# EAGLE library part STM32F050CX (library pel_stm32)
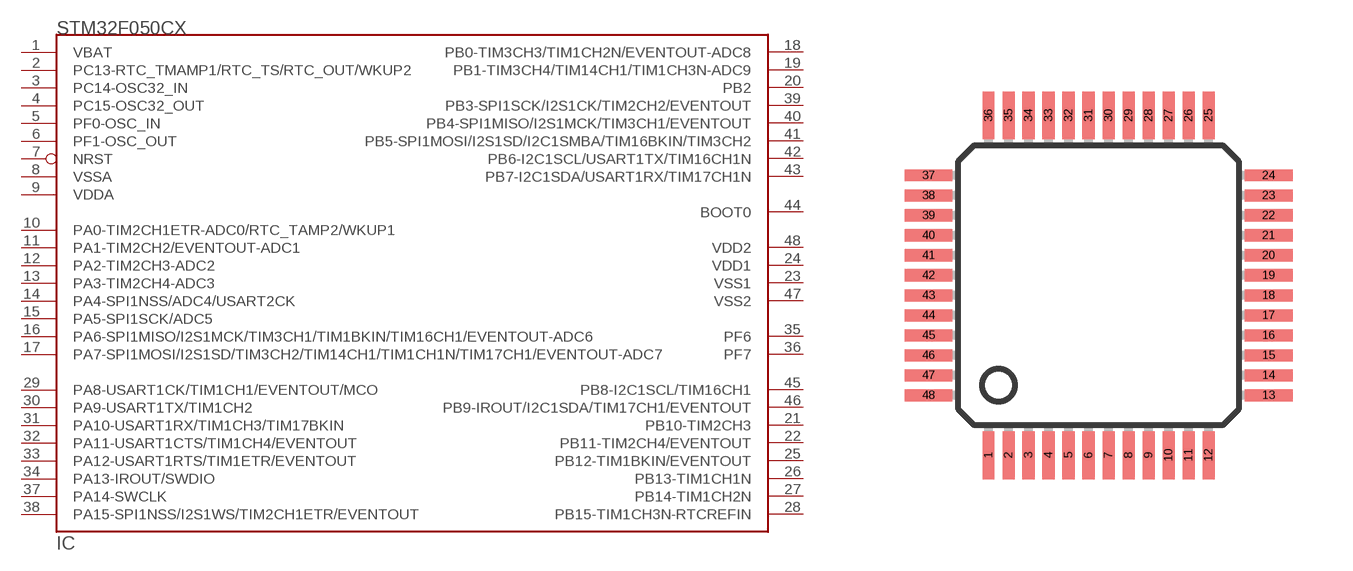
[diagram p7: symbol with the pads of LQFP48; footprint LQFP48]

Designator prefix IC

## STM32F050CX  [LQFP48]
1  VBAT  sup
2  PC13-RTC_TMAMP1/RTC_TS/RTC_OUT/WKUP2
3  PC14-OSC32_IN
4  PC15-OSC32_OUT
5  PF0-OSC_IN  in
6  PF1-OSC_OUT  out
7  NRST
8  VSSA  sup
9  VDDA  sup
10  PA0-TIM2CH1ETR-ADC0/RTC_TAMP2/WKUP1
11  PA1-TIM2CH2/EVENTOUT-ADC1
12  PA2-TIM2CH3-ADC2
13  PA3-TIM2CH4-ADC3
14  PA4-SPI1NSS/ADC4/USART2CK
15  PA5-SPI1SCK/ADC5
16  PA6-SPI1MISO/I2S1MCK/TIM3CH1/TIM1BKIN/TIM16CH1/EVENTOUT-ADC6
17  PA7-SPI1MOSI/I2S1SD/TIM3CH2/TIM14CH1/TIM1CH1N/TIM17CH1/EVENTOUT-ADC7
18  PB0-TIM3CH3/TIM1CH2N/EVENTOUT-ADC8
19  PB1-TIM3CH4/TIM14CH1/TIM1CH3N-ADC9
20  PB2
21  PB10-TIM2CH3
22  PB11-TIM2CH4/EVENTOUT
23  VSS1  sup
24  VDD1  sup
25  PB12-TIM1BKIN/EVENTOUT
26  PB13-TIM1CH1N
27  PB14-TIM1CH2N
28  PB15-TIM1CH3N-RTCREFIN
29  PA8-USART1CK/TIM1CH1/EVENTOUT/MCO
30  PA9-USART1TX/TIM1CH2
31  PA10-USART1RX/TIM1CH3/TIM17BKIN
32  PA11-USART1CTS/TIM1CH4/EVENTOUT
33  PA12-USART1RTS/TIM1ETR/EVENTOUT
34  PA13-IROUT/SWDIO
35  PF6  sup
36  PF7  sup
37  PA14-SWCLK
38  PA15-SPI1NSS/I2S1WS/TIM2CH1ETR/EVENTOUT
39  PB3-SPI1SCK/I2S1CK/TIM2CH2/EVENTOUT
40  PB4-SPI1MISO/I2S1MCK/TIM3CH1/EVENTOUT
41  PB5-SPI1MOSI/I2S1SD/I2C1SMBA/TIM16BKIN/TIM3CH2
42  PB6-I2C1SCL/USART1TX/TIM16CH1N
43  PB7-I2C1SDA/USART1RX/TIM17CH1N
44  BOOT0  in
45  PB8-I2C1SCL/TIM16CH1
46  PB9-IROUT/I2C1SDA/TIM17CH1/EVENTOUT
47  VSS2  sup
48  VDD2  sup

## Footprint LQFP48 (pad centres in mm)
Based on STM PCB layout recomendations.
smd 0.3 x 1.2: 1 -2.75,-4.25; 2 -2.25,-4.25; 3 -1.75,-4.25; 4 -1.25,-4.25; 5 -0.75,-4.25; 6 -0.25,-4.25; 7 0.25,-4.25; 8 0.75,-4.25; 9 1.25,-4.25; 10 1.75,-4.25; 11 2.25,-4.25; 12 2.75,-4.25; 25 2.75,4.25; 26 2.25,4.25; 27 1.75,4.25; 28 1.25,4.25; 29 0.75,4.25; 30 0.25,4.25; 31 -0.25,4.25; 32 -0.75,4.25; 33 -1.25,4.25; 34 -1.75,4.25; 35 -2.25,4.25; 36 -2.75,4.25
smd 1.2 x 0.3: 13 4.25,-2.75; 14 4.25,-2.25; 15 4.25,-1.75; 16 4.25,-1.25; 17 4.25,-0.75; 18 4.25,-0.25; 19 4.25,0.25; 20 4.25,0.75; 21 4.25,1.25; 22 4.25,1.75; 23 4.25,2.25; 24 4.25,2.75; 37 -4.25,2.75; 38 -4.25,2.25; 39 -4.25,1.75; 40 -4.25,1.25; 41 -4.25,0.75; 42 -4.25,0.25; 43 -4.25,-0.25; 44 -4.25,-0.75; 45 -4.25,-1.25; 46 -4.25,-1.75; 47 -4.25,-2.25; 48 -4.25,-2.75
